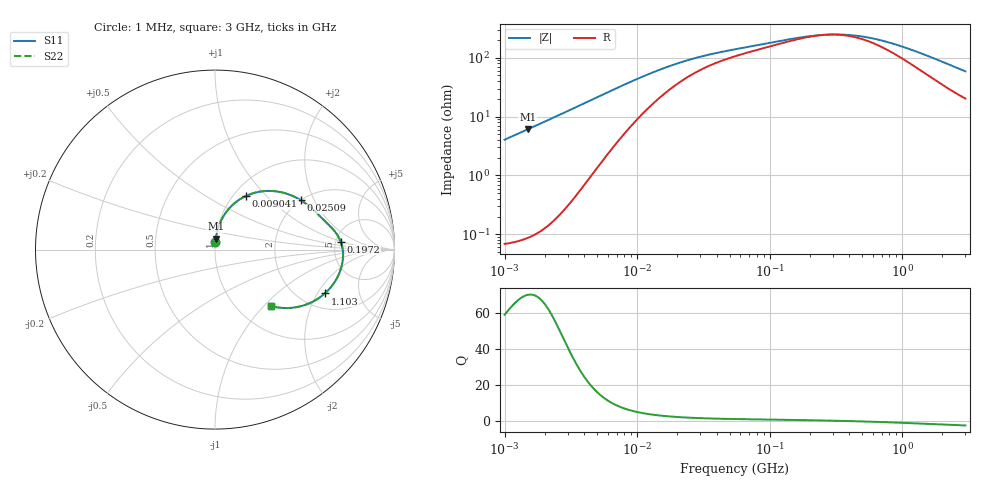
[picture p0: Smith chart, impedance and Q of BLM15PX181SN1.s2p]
! BLM15PX181SN1
# Hz S RI R 50
!Freq.(Hz) S11(Real) S11(Imag) S21(Real) S21(Imag) S12(Real) S12(Imag) S22(Real) S22(Imag)
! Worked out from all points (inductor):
!   401 points, 1 MHz to 3 GHz, reference 50 ohm
!   read as one part in series: L = 646 nH near 1.041 MHz
!   highest Q = 70 at 1.492 MHz (marker M1), where L = 648 nH
!   self-resonance near 273.7 MHz
!   S11 on the Smith chart (normalised r, x): 1 MHz: 1.00, +0.08; 9.041 MHz: 1.14, +0.78; 25.09 MHz: 1.99, +1.58; 197.2 MHz: 5.52, +0.98; 1.103 GHz: 2.69, -2.32; 3 GHz: 1.41, -1.10
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1000000  0.00232 0.0404  0.9977 -0.0404  0.9977 -0.0404  0.00232 0.0404
1492300  0.00453 0.0604  0.9955 -0.0604  0.9955 -0.0604  0.00453 0.0604
2461366  0.012 0.1  0.988 -0.1  0.988 -0.1  0.012 0.1
3823119  0.0307 0.1547  0.9693 -0.1547  0.9693 -0.1547  0.0307 0.1547
6058321  0.0825 0.2332  0.9175 -0.2332  0.9175 -0.2332  0.0825 0.2332
9040831  0.1742 0.2997  0.8258 -0.2997  0.8258 -0.2997  0.1742 0.2997
1.149534e7  0.2487 0.3227  0.7513 -0.3227  0.7513 -0.3227  0.2487 0.3227
1.461624e7  0.3279 0.326  0.6721 -0.326  0.6721 -0.326  0.3279 0.326
2.509235e7  0.4773 0.2756  0.5227 -0.2756  0.5227 -0.2756  0.4773 0.2756
3.526298e7  0.5386 0.2299  0.4614 -0.2299  0.4614 -0.2299  0.5386 0.2299
5.477226e7  0.5926 0.1785  0.4074 -0.1785  0.4074 -0.1785  0.5926 0.1785
1.971969e8  0.7 0.0449  0.3 -0.0449  0.3 -0.0449  0.7 0.0449
2.094008e8  0.7029 0.037  0.2971 -0.037  0.2971 -0.037  0.7029 0.037
2.942768e8  0.7128 -0.0105  0.2872 0.0105  0.2872 0.0105  0.7128 -0.0105
4.0536e8  0.7118 -0.06  0.2882 0.06  0.2882 0.06  0.7118 -0.06
5.583748e8  0.699 -0.1148  0.301 0.1148  0.301 0.1148  0.699 -0.1148
8.005644e8  0.6653 -0.1826  0.3347 0.1826  0.3347 0.1826  0.6653 -0.1826
1.10276e9  0.6118 -0.2442  0.3882 0.2442  0.3882 0.2442  0.6118 -0.2442
1.430499e9  0.5489 -0.2879  0.4511 0.2879  0.4511 0.2879  0.5489 -0.2879
1.893158e9  0.464 -0.3187  0.536 0.3187  0.536 0.3187  0.464 -0.3187
2.359433e9  0.3906 -0.3256  0.6094 0.3256  0.6094 0.3256  0.3906 -0.3256
3e9  0.3126 -0.3146  0.6874 0.3146  0.6874 0.3146  0.3126 -0.3146
